FUNCTION_BLOCK MOTORBLOCK
VAR_INPUT
	inputPointer :POINTER TO REAL;
END_VAR
VAR_OUTPUT
END_VAR
VAR	
	initDone : BOOL:= FALSE; 
	realMotorSpeed : REAL;
END_VAR


IF NOT initDone THEN
	inputPointer := ADR(realMotorSpeed);
	realMotorSpeed := 123.04; // default value
	initDone:= TRUE;
END_IF

IF inputPointer <> NULL THEN
inputPointer^:=realMotorSpeed; //new value is set after reading from the HW (not shown)
END_IF

END_FUNCTION_BLOCK
